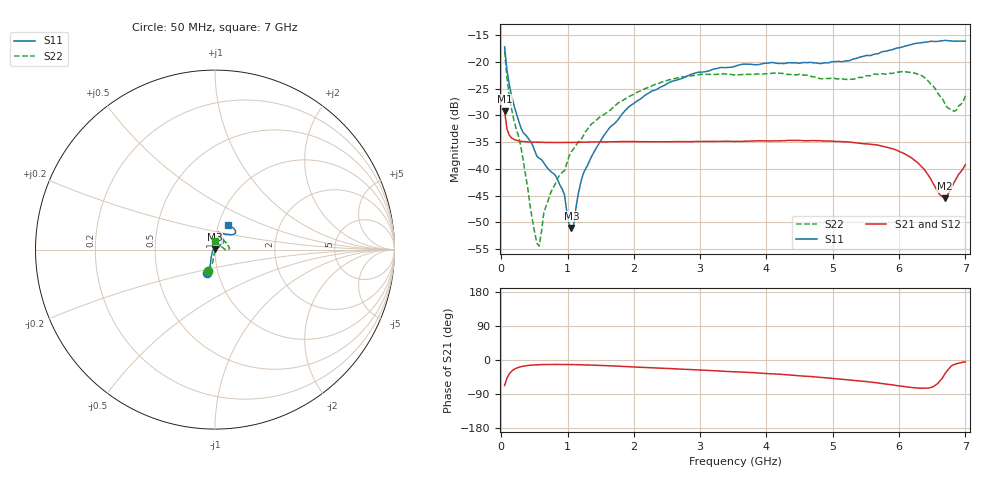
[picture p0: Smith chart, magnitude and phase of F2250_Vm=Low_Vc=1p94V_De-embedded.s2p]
! Integrated Device Technology
! Corporate Headquarters
! 6024 Silver Creek Valley Road
! San Jose, CA 95138  USA
! Phone:  1-408-284-8200
! Toll Free:  1-800-223-1366
! Webpage:  http://www.idt.com/
! Timing and RF Division
! 515 Groton Road, Suite 102
! Westford, MA 01886-6024
! Device:  F2250
! Description: Voltage Variable RF Attenuator
! Frequency:  50.0 -  6000.00 MHz
! Package:  3x3 mm Thin QFN Plastic Package: 16 pin
! Ports:  2 RF, 3 DC
!  Pin  1  = GND
!  Pin  2  = NC
!  Pin  3  = RF1  = Port 1
!  Pin  4  = NC
!  Pin  5  = GND
!  Pin  6  = GND
!  Pin  7  = GND
!  Pin  8  = GND
!  Pin  9  = NC
!  Pin 10  = RF2  = Port 2
!  Pin 11  = NC
!  Pin 12  = GND
!  Pin 13  = GND
!  Pin 14  = VCNTRL
!  Pin 15  = VDD
!  Pin 16  = VMODE
! Vcntrl:  1.940 Volts
! Vmode:  +0.000 Volts
! Vdd:  +3.30  Volts
! Current:  1.183 mA
! Data:  The device was measured on a the F2250 evaluation board which has
!  individual transmission lines to the RF pins.  Data was collected
!  using a calibrated network analyzer.  The evaluation board was
!  de-embedded using a TRL calibration technique.
!  The reference plane is the edge of the package pin.
! Misc:  SN 10
!  Action Tracker AT0258
! Date Measured:  2014-11-26
! Date:  2015-10-15  MJV
! Note:
!  Integrated Device Technology supplies this data as a sample of measured
!  data at the package pin for this product.  Your particular data for this
!  product may vary.
!  Data was taken at 25 degrees C.
!  Integrated Device Technology reserves the right to change this data at anytime.
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# GHz S dB R 50
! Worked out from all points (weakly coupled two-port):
!   201 points, 50 MHz to 7 GHz, reference 50 ohm
!   highest |S21| = -29.19 dB at 50 MHz (marker M1); lowest = -45.5 dB at 6.687 GHz (marker M2)
!   lowest |S11| = -51.0 dB at 1.058 GHz (marker M3), VSWR 1.01, Z = 49.9 + j0.24 ohm
!   |S11| at or under -10 dB: start of sweep to end of sweep
!   |S22| runs from -54.4 to -18.1 dB; largest |S21 - S12| = 6.2e-05
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0.05  -17.18 -108.6  -29.19 -67.4  -29.19 -67.4  -18.07 -106.9
0.1195  -24.20 -111.7  -33.67 -36.8  -33.68 -36.8  -26.24 -100.4
0.22375  -29.51 -121.9  -34.65 -21.9  -34.65 -21.9  -32.49 -100.0
0.29325  -32.22 -127.5  -34.83 -17.8  -34.83 -17.8  -35.67 -93.2
0.5365  -37.62 -155.1  -35.02 -12.7  -35.02 -12.7  -53.86 -42.4
0.57125  -38.02 -160.2  -35.03 -12.4  -35.03 -12.4  -54.45 -13.0
0.64075  -38.86 -160.9  -35.05 -12.0  -35.05 -12.1  -48.27 21.9
0.745  -40.49 -174.7  -35.06 -11.8  -35.06 -11.8  -44.46 32.2
0.91875  -43.76 157.9  -35.07 -11.8  -35.07 -11.8  -40.64 35.5
1.05775  -51.03 120.9  -35.06 -12.0  -35.06 -12.0  -36.77 39.9
1.0925  -50.51 87.5  -35.05 -12.1  -35.05 -12.1  -36.23 38.0
1.162  -44.58 55.4  -35.04 -12.3  -35.04 -12.3  -35.01 33.5
1.2315  -41.06 43.7  -35.01 -12.6  -35.01 -12.6  -33.93 30.7
1.6485  -32.10 41.6  -34.94 -15.4  -34.94 -15.4  -28.95 36.1
2.37825  -24.87 47.2  -34.91 -21.3  -34.91 -21.3  -24.01 41.4
3.525  -20.81 72.4  -34.86 -31.0  -34.87 -31.0  -22.43 66.1
4.7065  -20.18 72.3  -34.71 -44.2  -34.70 -44.2  -22.78 67.2
5.85325  -17.82 40.4  -36.08 -64.6  -36.09 -64.7  -22.13 14.3
6.33975  -16.40 40.9  -39.62 -74.5  -39.63 -74.5  -22.57 0.1
6.68725  -15.99 48.8  -45.50 -37.4  -45.50 -37.2  -27.70 20.5
6.82625  -16.14 53.5  -42.60 -12.4  -42.55 -12.4  -29.23 52.1
7  -16.13 63.2  -39.21 -5.0  -39.17 -5.1  -26.33 89.8
